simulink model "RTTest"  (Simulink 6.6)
settings: Solver=FixedStepDiscrete  StartTime=0.0  StopTime=inf  RelTol=1e-3
PreLoadFcn:
  | scramInitialize
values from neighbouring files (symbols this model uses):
  node = completenodestruct(node)    [scramInitialize.m]
  nTbl = 6    [scramInitialize.m]
  samplePeriod = 1/1024    (= 0.0009765625)    [scramInitialize.m]    (also in viewer.m = eval(getHeaderValue(header, 'DELTA_T')))
undefined symbols (not defined in the file or in its folder): DiscIntNeverNeededParam, Flat
libraries: xpcsystranlib x3, xpclib x3, simulink x1

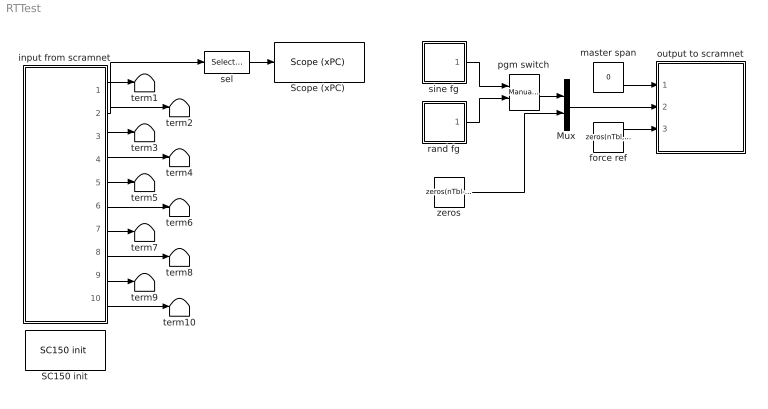
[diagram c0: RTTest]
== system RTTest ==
  Mux : Mux  Inputs=2
  SC150 init : xpcsystranlib/Shared Memory/SC150 init   node=node  pci=-1
  "Scope (xPC) " : xpclib/Misc./Scope (xPC)   SystemSampleTime=-1  scopeno=1  scopetype=Target  autostart=on  viewmode=Graphical redraw  formatstr='%15.6f'  grid=on  ylimits=[0,0]  nosamples=1024  noprepostsamples=0  interleave=1  triggermode=FreeRun  triggersignal=1  triggerlevel=0.0  triggerslope=Either  triggerscope=1  triggersample=0  filename=data.dat  mode=Lazy  writesize=512  autorestart=off
  force ref : Constant  Value=zeros(nTbl, 1)
  input from scramnet : Subsystem
  master span : Constant  Value=0
  output to scramnet : Subsystem
  pgm switch : simulink/Signal Routing/Manual Switch  SystemSampleTime=-1  sw=1  action=0  varsize=off
  rand fg : Subsystem  mask(Random Function Generator){shape=Flat, ampl=0.05, minFreq=0, maxFreq=10, spanInterval=1, samplePeriod=samplePeriod, showFRF=off}
      mask prompts: ampl "RMS amplitude"; minFreq "Minimum frequency (Hz)"; maxFreq "Maximum frequency (Hz)"; spanInterval "Span interval (sec)"; samplePeriod "Sample period (sec)"; showFRF "Show filter frequency response"
      mask init:
      | fsamp	= 1 / samplePeriod;
      | 
      | % design shaping filter
      | switch (shape)
      | 	case '1/F^2'	% 1/f^2 (two-pole lowpass)
      | 		% Note: Has unity amplitude at minFreq, then
      | 		% decreases at -40db per decade up to maxFreq.
      | 		minFreq = max(minFreq, 0.01*maxFreq);
      | 		k		= 0.1;
      | 		fpass	= k * minFreq;
      | 		alpha	= -exp(-2 * pi * fpass / fsamp);
      | 		a1		= 2 * alpha;
      | 		a2		= alpha^2;
      | 		b0		= (1/k)^2 * (1 + a1 + a2) * 0.25;
      | 		b1		= 2 * b0
      | 		b2		= b0
      | 		noiseBw = (minFreq / 3) * (1 - (minFreq / maxFreq)^3);
      | 	case '1/F'		% 1/f (one-pole lowpass)
      | 		% Note: Has unity amplitude at minFreq, then
      | 		% decreases at -20db per decade up to maxFreq.
      | 		minFreq = max(minFreq, 0.01*maxFreq);
      | 		k		= 0.1;
      | 		fpass	= k * minFreq;
      | 		alpha	= -exp(-2 * pi * fpass / fsamp);
      | 		a1		= alpha;
      | 		a2		= 0;
      | 		b0		= (1/k) * (1 + a1) * 0.5;
      | 		b1		= b0;
      | 		b2		= 0;
      | 		noiseBw = minFreq * (1 - (minFreq / maxFreq));
      | 	case 'Flat'		% flat
      | 		fpass	= maxFreq;
      | 		a1		= 0;
      | 		a2		= 0;
      | 		b0		= 1;
      | 		b1		= 0;
      | 		b2		= 0;
      | 		noiseBw = maxFreq - minFreq;
      | 	case 'F'		% f (single differentiator)
      | 		% Note:  A simple backward difference is a valid
      | 		% differentiator only up to about one half of nyquist.
      | 		% So we will select coefficients so that the slope,
      | 		% if extrapolated, would reach unity gain at nyquist
      | 		% (in reality, the gain will fall short of unity).
      | 		% These coefficients will be experimentally determined.
      | 		a1		= 0;
      | 		a2		= 0;
      | 		b0		= 0.33;
      | 		b1		= -b0;
      | 		b2		= 0;
      | 		noiseBw	= (4/3) * (maxFreq*(maxFreq/fsamp)^2 - minFreq*(minFreq/fsamp)^2);
      | 	case 'F^2'		% f^2 (double differentiator)
      | 		% Note:  See note above.
      | 		a1		= 0;
      | 		a2		= 0;
      | 		b0		= (0.33)^2;
      | 		b1		= -2 * b0;
      | 		b2		= b0;
      | 		noiseBw = (16/5) * (maxFreq*(maxFreq/fsamp)^4 - minFreq*(minFreq/fsamp)^4);
      | end
      | aSpf = [1 a1 a2];
      | bSpf = [b0 b1 b2];
      | peakAmpl = ampl * sqrt(3) * sqrt(max(0.5*fsamp/noiseBw, 1));
      | 
      | % design bandlimiting filter
      | fpassU	= maxFreq;
      | fstopU	= fpassU * 1.25;
      | fpassL	= min(minFreq, fpassU-0.001);
      | fstopL	= fpassL * 0.5;
      | rpass	= 0.01;
      | rstop	= 0.01;
      | rpassDB	= -20*log10(1-rpass);
      | rstopDB	= -20*log10(rstop);
      | bHpf	= [1];
      | aHpf	= [1];
      | bLpf	= [1];
      | aLpf	= [1];
      | if fpassL == 0
      | 		if fstopU < 0.5 * fsamp		% lowpass
      | 			[n, wn]	= ellipord(2*fpassU/fsamp, 2*fstopU/fsamp, rpassDB, rstopDB);
      | 			[bLpf, aLpf] = ellip(n, rpassDB, rstopDB, wn, 'low');
      | 		end
      | else
      | 		if fstopU < 0.5 * fsamp		% bandpass (implemented as series HP & LP)
      | 			rpassDB = rpassDB / 2;
      | 			[n, wn]	= ellipord(2*fpassU/fsamp, 2*fstopU/fsamp, rpassDB, rstopDB);
      | 			[bLpf, aLpf] = ellip(n, rpassDB, rstopDB, wn, 'low');
      | 			[n, wn]	= ellipord(2*fpassL/fsamp, 2*fstopL/fsamp, rpassDB, rstopDB);
      | 			[bHpf, aHpf] = ellip(n, rpassDB, rstopDB, wn, 'high');
      | 		else						% highpass
      | 			[n, wn]	= ellipord(2*fpassU/fsamp, 2*fstopU/fsamp, rpassDB, rstopDB);
      | 			[bHpf, aHpf] = ellip(n, rpassDB, rstopDB, wn, 'high');
      | 		end	
      | end
      | if showFRF
      | 	f     = linspace(0, fsamp/4, 8192);
      | 	tfSpf = freqz(bSpf, aSpf, f, fsamp);
      | 	tfLpf = freqz(bLpf, aLpf, f, fsamp);
      | 	tfHpf = freqz(bHpf, aHpf, f, fsamp);
      | 	plot(f, 20*log10(peakAmpl*abs(tfSpf.*tfLpf.*tfHpf)));
      | 	title('Filter Frequency Response');
      | 	ylabel('dB');
      | 	xlabel('Hz');
      | end
  sel : Selector  IndexOptions=Index vector (dialog)  Indices=1  OutputSizes=1
  sine fg : Subsystem  mask(Sine Function Generator){ampl=0.1, freq=5, spanInterval=1, samplePeriod=samplePeriod}
      mask prompts: ampl "Amplitude"; freq "Frequency (Hz)"; spanInterval "Span interval (sec)"; samplePeriod "Sample period (sec)"
  term{1..10} (10 alike) : Terminator
  zeros : Constant  Value=zeros(nTbl-1, 1)
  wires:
  master span/1 -> output to scramnet/1(master span)
  input from scramnet/1(master span) -> term1/1
  input from scramnet/2(displ ref) -> term2/1, sel/1
  input from scramnet/3(veloc ref) -> term3/1
  input from scramnet/4(force ref) -> term4/1
  sel/1 -> "Scope (xPC) "/1
  sine fg/1(out) -> pgm switch/1
  rand fg/1(out) -> pgm switch/2
  pgm switch/1 -> Mux/1
  zeros/1 -> Mux/2
  Mux/1 -> output to scramnet/2(displ ref)
  force ref/1 -> output to scramnet/3(force ref)
  input from scramnet/5(displ fbk) -> term5/1
  input from scramnet/6(veloc fbk) -> term6/1
  input from scramnet/7(force fbk) -> term7/1
  input from scramnet/8(comp fbk) -> term8/1
  input from scramnet/9(press fbk) -> term9/1
  input from scramnet/10(user adcs) -> term10/1

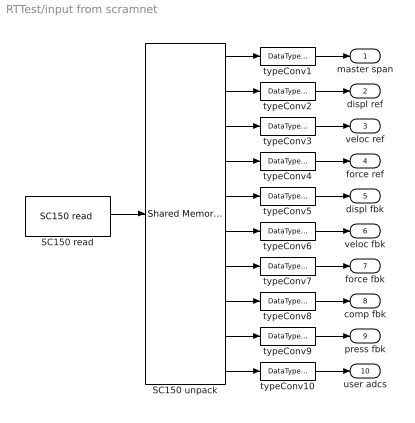
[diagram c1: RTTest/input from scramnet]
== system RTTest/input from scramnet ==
  SC150 read : xpcsystranlib/Shared Memory/SC150 read   partition=node.Partitions(4:end)  errorport=off  ts=samplePeriod  pci=-1
  SC150 unpack : xpclib/Shared Memory/Shared Memory Unpack   partition=node.Partitions(4:end)
  typeConv{1..10} (10 alike) : DataTypeConversion  OutDataTypeMode=double
  master span : Outport
  displ ref : Outport  Port=2
  veloc ref : Outport  Port=3
  force ref : Outport  Port=4
  displ fbk : Outport  Port=5
  veloc fbk : Outport  Port=6
  force fbk : Outport  Port=7
  comp fbk : Outport  Port=8
  press fbk : Outport  Port=9
  user adcs : Outport  Port=10
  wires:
  SC150 read/1 -> SC150 unpack/1
  typeConv1/1 -> master span/1
  typeConv2/1 -> displ ref/1
  typeConv3/1 -> veloc ref/1
  typeConv4/1 -> force ref/1
  SC150 unpack/1 -> typeConv1/1
  SC150 unpack/2 -> typeConv2/1
  SC150 unpack/3 -> typeConv3/1
  SC150 unpack/4 -> typeConv4/1
  SC150 unpack/5 -> typeConv5/1
  SC150 unpack/6 -> typeConv6/1
  typeConv5/1 -> displ fbk/1
  typeConv6/1 -> veloc fbk/1
  SC150 unpack/7 -> typeConv7/1
  SC150 unpack/8 -> typeConv8/1
  SC150 unpack/9 -> typeConv9/1
  SC150 unpack/10 -> typeConv10/1
  typeConv10/1 -> user adcs/1
  typeConv9/1 -> press fbk/1
  typeConv8/1 -> comp fbk/1
  typeConv7/1 -> force fbk/1

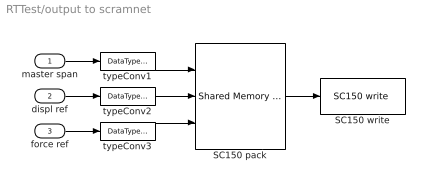
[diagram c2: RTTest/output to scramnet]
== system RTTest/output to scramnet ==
  master span : Inport
  displ ref : Inport  Port=2
  force ref : Inport  Port=3
  SC150 pack : xpclib/Shared Memory/Shared Memory Pack   partition=node.Partitions(1:3)
  SC150 write : xpcsystranlib/Shared Memory/SC150 write   partition=node.Partitions(1:3)  errorport=off  ts=samplePeriod  pci=-1
  typeConv1 : DataTypeConversion  OutDataTypeMode=single
  typeConv2 : DataTypeConversion  OutDataTypeMode=single
  typeConv3 : DataTypeConversion  OutDataTypeMode=single
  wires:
  master span/1 -> typeConv1/1
  displ ref/1 -> typeConv2/1
  SC150 pack/1 -> SC150 write/1
  typeConv1/1 -> SC150 pack/1
  typeConv2/1 -> SC150 pack/2
  force ref/1 -> typeConv3/1
  typeConv3/1 -> SC150 pack/3

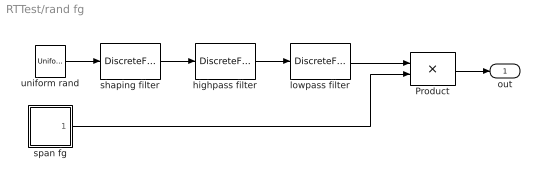
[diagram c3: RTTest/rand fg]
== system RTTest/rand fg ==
  Product : Product
  highpass filter : DiscreteFilter  Numerator=bHpf  Denominator=aHpf  SampleTime=samplePeriod
  lowpass filter : DiscreteFilter  Numerator=bLpf  Denominator=aLpf  SampleTime=samplePeriod
  shaping filter : DiscreteFilter  Numerator=bSpf  Denominator=aSpf  SampleTime=samplePeriod
  span fg : Subsystem  mask{spanInterval=spanInterval, samplePeriod=samplePeriod}
      mask prompts: spanInterval "Span interval (sec)"; samplePeriod "Sample period (sec)"
  uniform rand : UniformRandomNumber  Minimum=-peakAmpl  Maximum=peakAmpl  SampleTime=samplePeriod
  out : Outport
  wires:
  lowpass filter/1 -> Product/1
  highpass filter/1 -> lowpass filter/1
  shaping filter/1 -> highpass filter/1
  uniform rand/1 -> shaping filter/1
  Product/1 -> out/1
  span fg/1(out) -> Product/2

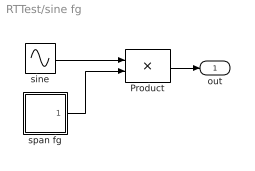
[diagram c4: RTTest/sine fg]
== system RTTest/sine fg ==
  Product : Product
  sine : Sin  Amplitude=ampl  Frequency=2 * pi * freq  SampleTime=samplePeriod
  span fg : Subsystem  mask{spanInterval=spanInterval, samplePeriod=samplePeriod}
      mask prompts: spanInterval "Span interval (sec)"; samplePeriod "Sample period (sec)"
  out : Outport
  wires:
  span fg/1(out) -> Product/2
  sine/1 -> Product/1
  Product/1 -> out/1

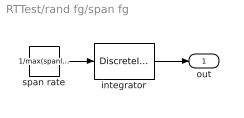
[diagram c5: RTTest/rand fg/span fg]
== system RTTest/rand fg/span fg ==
  integrator : DiscreteIntegrator  SampleTime=samplePeriod  LimitOutput=on  UpperSaturationLimit=1  LowerSaturationLimit=0  ICPrevOutput=DiscIntNeverNeededParam  ICPrevScaledInput=DiscIntNeverNeededParam
  span rate : Constant  Value=1/max(spanInterval,samplePeriod)  SampleTime=samplePeriod
  out : Outport
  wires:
  integrator/1 -> out/1
  span rate/1 -> integrator/1

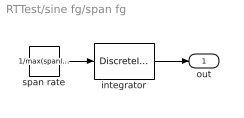
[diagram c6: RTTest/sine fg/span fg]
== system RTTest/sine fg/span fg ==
  integrator : DiscreteIntegrator  SampleTime=samplePeriod  LimitOutput=on  UpperSaturationLimit=1  LowerSaturationLimit=0  ICPrevOutput=DiscIntNeverNeededParam  ICPrevScaledInput=DiscIntNeverNeededParam
  span rate : Constant  Value=1/max(spanInterval,samplePeriod)  SampleTime=samplePeriod
  out : Outport
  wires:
  integrator/1 -> out/1
  span rate/1 -> integrator/1
